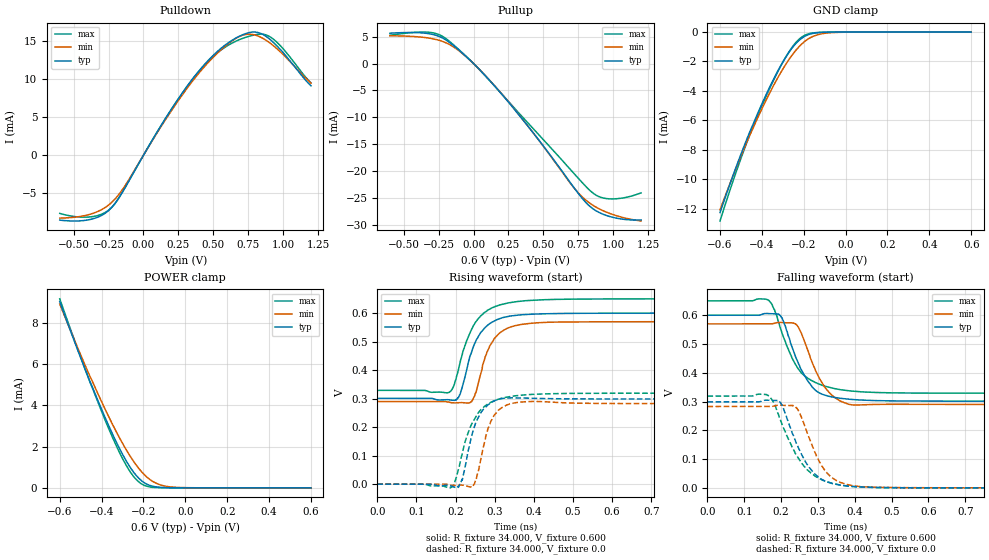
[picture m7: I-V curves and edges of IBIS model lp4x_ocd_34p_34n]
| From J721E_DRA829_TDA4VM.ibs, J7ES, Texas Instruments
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|   Model lp4x_ocd_34p_34n
[Model] lp4x_ocd_34p_34n
Model_type I/O
Polarity   Non-Inverting
Enable   Active-High
Vinl =  0.0V
Vinh =  0.900V
Vmeas =  0.600V
C_comp   1.578pF   1.388pF   1.856pF
[Model Spec]
Vinh   0.900V   0.900V   0.900V
Vinl   0.0V   0.0V   0.0V
Vmeas   0.600V   NA   NA
[Temperature Range]   25.000   0.125k   -40.000
[Voltage Range]   0.600V   0.570V   0.650V
[Pullup Reference]   0.600V   0.570V   0.650V
[Pulldown Reference]   0.0V   0.0V   0.0V
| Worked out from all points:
|   slope of the pulldown table from 0 to 0.09 V, typ, clamps not added: 32 ohm
|   slope of the pullup table from 0 to 0.09 V, typ, clamps not added: 37.2 ohm
|   GND clamp passes 1 mA (typ) near -0.25 V on its own axis
|   POWER clamp passes 1 mA (typ) near -0.26 V on its own axis
|   rising waveform, R_fixture 34.000, V_fixture 0.600: 20-80 % time 48.6ps typ, 44.5ps min, 55.8ps max; typ from 0.301 V to 0.6 V
|   rising waveform, R_fixture 34.000, V_fixture 0.0: 20-80 % time 35.8ps typ, 32.7ps min, 51.1ps max; typ from 0 V to 0.299 V
|   falling waveform, R_fixture 34.000, V_fixture 0.600: 20-80 % time 61.4ps typ, 58.7ps min, 69.7ps max; typ from 0.6 V to 0.301 V
|   falling waveform, R_fixture 34.000, V_fixture 0.0: 20-80 % time 66.8ps typ, 60.4ps min, 77.9ps max; typ from 0.299 V to 0 V
[Pulldown]
|Voltage   I(typ)   I(min)   I(max)
-600mV    -8.529mA   -8.268mA   -7.651mA
-392mV    -8.486mA   -7.808mA   -8.124mA
-240mV    -7.101mA   -6.4mA     -7.068mA
-145mV    -4.679mA   -4.36mA    -4.656mA
120mV     3.725mA    3.598mA    3.704mA
328mV     9.463mA    9.189mA    9.418mA
499mV     13.12mA    12.87mA    12.97mA
669mV     15.48mA    15.43mA    15.05mA
802mV     16.19mA    15.79mA    15.84mA
897mV     15.37mA    14.88mA    15.67mA
992mV     13.67mA    13.4mA     14.18mA
1.2V      9.119mA    9.474mA    9.501mA
[Pullup]
|Voltage   I(typ)   I(min)   I(max)
-600mV    5.66mA     5.174mA    5.283mA
-297mV    5.453mA    4.649mA    5.756mA
-221mV    4.75mA     4.115mA    5.046mA
-107mV    2.553mA    2.43mA     2.645mA
44.21mV   -1.16mA    -1.151mA   -1.182mA
234mV     -6.678mA   -6.632mA   -6.587mA
480mV     -14.66mA   -14.7mA    -13.6mA
726mV     -23.32mA   -23.33mA   -20.64mA
859mV     -27.08mA   -26.43mA   -24.17mA
916mV     -27.91mA   -27.24mA   -24.92mA
992mV     -28.58mA   -28.04mA   -25.18mA
1.2V      -29.1mA    -29.29mA   -24.06mA
[GND_clamp]
|Voltage   I(typ)   I(min)   I(max)
-600mV    -12.26mA   -12.07mA   -12.83mA
-535mV    -9.631mA   -9.657mA   -9.999mA
-483mV    -7.674mA   -7.84mA    -7.926mA
-457mV    -6.749mA   -6.974mA   -6.957mA
-378mV    -4.198mA   -4.571mA   -4.306mA
-326mV    -2.705mA   -3.156mA   -2.747mA
-287mV    -1.735mA   -2.22mA    -1.722mA
-248mV    -949.8uA   -1.424mA   -887.7uA
-209mV    -414uA     -806.5uA   -336.6uA
-157mV    -95.46uA   -302uA     -61.65uA
-78.26mV  -9.124uA   -53.02uA   -8.177uA
600mV     0A         0A         0A
[POWER_clamp]
|Voltage   I(typ)   I(min)   I(max)
-600mV    9.037mA    8.928mA    9.175mA
-457mV    5.197mA    5.441mA    5.166mA
-352mV    2.698mA    3.164mA    2.544mA
-313mV    1.878mA    2.4mA      1.683mA
-274mV    1.164mA    1.707mA    946.8uA
-248mV    770.5uA    1.297mA    560.4uA
-222mV    461.8uA    938.3uA    283.7uA
-196mV    246uA      638.8uA    120.5uA
-157mV    79.32uA    316.3uA    23.58uA
-117mV    22.65uA    136.3uA    6.085uA
-78.26mV  6.713uA    54.46uA    1.894uA
600mV     0A         0A         0A
[Ramp]
| variable   typ   min   max
dV/dt_r   0.179/35.452p   0.170/32.474p   0.191/51.695p
dV/dt_f   0.180/61.671p   0.168/58.656p   0.193/68.830p
R_load = 34.000
[Rising Waveform]
R_fixture= 34.000
V_fixture= 0.600
V_fixture_min= 0.570
V_fixture_max= 0.650
|time   V(typ)   V(min)   V(max)
0s        301.1mV    289.8mV    329mV
184ps     295.9mV    287.3mV    322.1mV
197ps     294.4mV    284.9mV    350.5mV
211ps     313.5mV    286mV      424.8mV
237ps     449.6mV    285.9mV    531.4mV
252ps     503.6mV    320.9mV    569.9mV
263ps     529.7mV    381.7mV    589mV
298ps     571.9mV    509.3mV    621.1mV
381ps     595.3mV    562.6mV    643.8mV
3ns       600mV      569.9mV    650mV
[Rising Waveform]
R_fixture= 34.000
V_fixture= 0.0
V_fixture_min= 0.0
V_fixture_max= 0.0
|time   V(typ)   V(min)   V(max)
0s        30.9uV     160.2uV    31.06uV
191ps     -7.556mV   -4.113mV   -9.606mV
217ps     14.25mV    -3.308mV   107.5mV
244ps     183.8mV    -8.326mV   218.4mV
252ps     217.8mV    12.88mV    236.7mV
266ps     253.9mV    99.52mV    263mV
294ps     288.8mV    232mV      290.1mV
329ps     301.9mV    276.9mV    304.8mV
381ps     301.8mV    289.3mV    313.7mV
3ns       298.9mV    282.8mV    319.1mV
[Falling Waveform]
R_fixture= 34.000
V_fixture= 0.600
V_fixture_min= 0.570
V_fixture_max= 0.650
|time   V(typ)   V(min)   V(max)
0s        600mV      569.9mV    650mV
167ps     605.7mV    569.9mV    651.1mV
182ps     604.8mV    572mV      619.5mV
202ps     592.1mV    574.7mV    539.2mV
239ps     456.4mV    570.2mV    429.4mV
274ps     368.2mV    471.6mV    379.7mV
317ps     322.9mV    352.1mV    354.4mV
360ps     311.3mV    302.1mV    341.3mV
400ps     306.5mV    287.8mV    335.3mV
3ns       301.1mV    289.8mV    329mV
[Falling Waveform]
R_fixture= 34.000
V_fixture= 0.0
V_fixture_min= 0.0
V_fixture_max= 0.0
|time   V(typ)   V(min)   V(max)
0s        298.9mV    282.8mV    319.1mV
163ps     304.7mV    282.8mV    322.9mV
177ps     303.5mV    283.3mV    303.2mV
199ps     295.5mV    287.5mV    232.6mV
237ps     168.9mV    283.9mV    124.5mV
276ps     71.43mV    174.7mV    57.19mV
315ps     26.56mV    66.99mV    25.38mV
347ps     12.62mV    27.11mV    13.03mV
394ps     4.764mV    7.74mV     4.779mV
3ns       30.67uV    159.2uV    30.8uV
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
